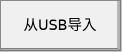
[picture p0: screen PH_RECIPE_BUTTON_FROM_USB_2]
VISUALIZATION PH_RECIPE_BUTTON_FROM_USB_2  // 122x52
VAR_IN_OUT
	RECIPE_CTRL_V2 : ST_RecipeCtrl_2;
END_VAR
    Button (0,0 120x50), "从USB导入", input disabled if: (RECIPE_CTRL_V2.sStatus.bBusy) <> 0, text list: 'TextList_Recipe', text index: 119
        p55702900: SEL(RECIPE_CTRL_V2.sCmd.bRecipeLoadFromUSB, 16#000000, 16#00FF00)
        tap RECIPE_CTRL_V2.sCmd.bRecipeLoadFromUSB
END_VISUALIZATION
